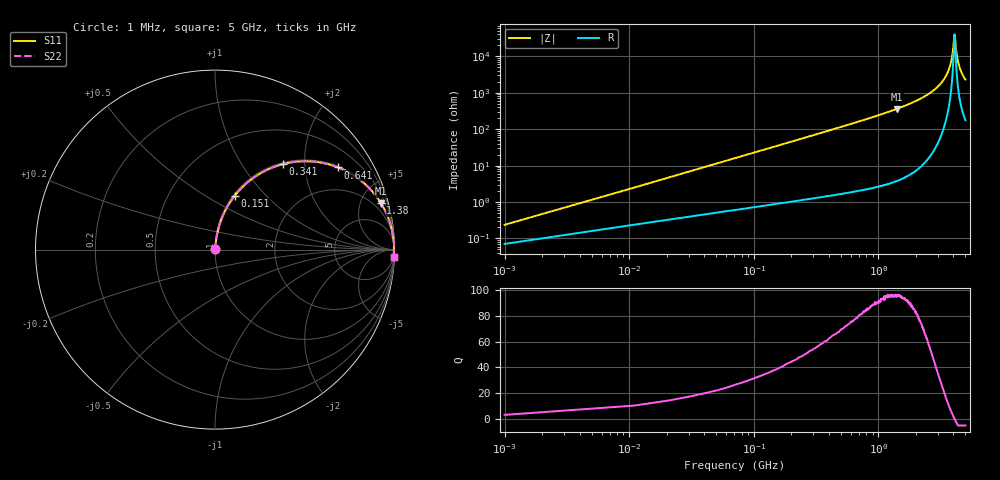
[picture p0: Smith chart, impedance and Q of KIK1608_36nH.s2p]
!version-2
!date-01.2022
!Series
# MHz S RI R 50
!Freq ReS11 ImS11 ReS21 ImS21 ReS12 ImS12 ReS22 ImS22
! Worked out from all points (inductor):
!   501 points, 1 MHz to 5 GHz, reference 50 ohm
!   read as one part in series: L = 36 nH near 21 MHz
!   highest Q = 95.9 at 1.4 GHz (marker M1), where L = 40.8 nH
!   self-resonance near 4.09 GHz
!   S11 on the Smith chart (normalised r, x): 1 MHz: 1.00, +0.00; 151 MHz: 1.02, +0.68; 341 MHz: 1.03, +1.55; 641 MHz: 1.04, +2.97; 1.38 GHz: 1.07, +7.05; 5 GHz: 5, -46
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1  0.000724 0.00226  0.9993 -0.00226  0.9993 -0.00226  0.000724 0.00226
31  0.00882 0.0692  0.9912 -0.0692  0.9912 -0.0692  0.00882 0.0692
41  0.013 0.0911  0.987 -0.0911  0.987 -0.0911  0.013 0.0911
81  0.0383 0.1751  0.9617 -0.1751  0.9617 -0.1751  0.0383 0.1751
151  0.111 0.3014  0.889 -0.3014  0.889 -0.3014  0.111 0.3014
341  0.3784 0.4764  0.6216 -0.4764  0.6216 -0.4764  0.3784 0.4764
641  0.6862 0.4576  0.3138 -0.4576  0.3138 -0.4576  0.6862 0.4576
841  0.795 0.3979  0.205 -0.3979  0.205 -0.3979  0.795 0.3979
1380  0.9232 0.2611  0.0768 -0.2611  0.0768 -0.2611  0.9232 0.2611
1400  0.9257 0.2571  0.0743 -0.2571  0.0743 -0.2571  0.9257 0.2571
1670  0.9516 0.2093  0.0484 -0.2093  0.0484 -0.2093  0.9516 0.2093
2510  0.9863 0.1082  0.0137 -0.1082  0.0137 -0.1082  0.9863 0.1082
3340  0.996 0.044  0.00397 -0.044  0.00397 -0.044  0.996 0.044
3630  0.9971 0.0259  0.00285 -0.0259  0.00285 -0.0259  0.9971 0.0259
3830  0.9975 0.0144  0.00251 -0.0144  0.00251 -0.0144  0.9975 0.0144
3960  0.9976 0.00718  0.00244 -0.00718  0.00244 -0.00718  0.9976 0.00718
4090  0.9975 0.000246  0.00249 -0.000246  0.00249 -0.000246  0.9975 0.000246
4120  0.9975 -0.00132  0.00251 0.00132  0.00251 0.00132  0.9975 -0.00132
4170  0.9974 -0.00391  0.00257 0.00391  0.00257 0.00391  0.9974 -0.00391
4280  0.9973 -0.0095  0.00273 0.0095  0.00273 0.0095  0.9973 -0.0095
4450  0.9969 -0.0179  0.0031 0.0179  0.0031 0.0179  0.9969 -0.0179
5000  0.9948 -0.043  0.00517 0.043  0.00517 0.043  0.9948 -0.043
